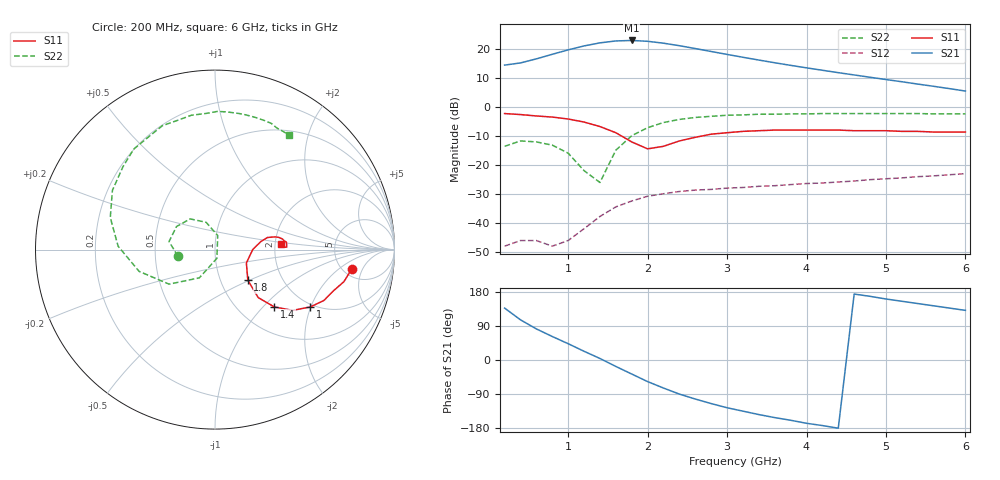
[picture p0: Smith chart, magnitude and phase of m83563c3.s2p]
!	MGA-83563 S PARAMETERS
!	Vd = 3 V L=4.7 nH  LAST UPDATED 10-15-97
# ghz	s ma r	50
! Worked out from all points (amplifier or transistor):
!   30 points, 200 MHz to 6 GHz, reference 50 ohm
!   highest |S21| = 22.9 dB at 1.8 GHz (marker M1)
!   |S21| within 3 dB of that: 1.036 GHz to 2.642 GHz (1.606 GHz wide, 87.3 % of centre)
!   unconditionally stable (mu >= 1): start of sweep to end of sweep
!   at 1.2 GHz: K = 3.89, MAG = 22.6 dB, |S12| = -41.9 dB
!   at 3.2 GHz: K = 1.07, MAG = 20.9 dB, |S12| = -27.7 dB
!   at 6 GHz: K = 1.46, MAG = 10.2 dB, |S12| = -23.0 dB
!   S11 on the Smith chart (normalised r, x): 200 MHz: 6.00, -3.16; 1 GHz: 1.91, -1.99; 1.4 GHz: 1.43, -1.16; 1.8 GHz: 1.35, -0.49; 6 GHz: 2.16, +0.16
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0.2  0.77 -8.0  5.26 137.0  0.004 56.0  0.21 -170.0
0.4  0.74 -14.0  5.74 106.0  0.005 42.0  0.26 170.0
0.6  0.7 -19.0  6.74 82.0  0.005 41.0  0.25 149.0
0.8  0.67 -25.0  8.08 62.0  0.004 59.0  0.22 129.0
1  0.62 -31.0  9.63 43.0  0.005 91.0  0.16 108.0
1.2  0.55 -38.0  11.26 23.0  0.008 107.0  0.08 79.0
1.4  0.46 -44.0  12.72 4.0  0.013 109.0  0.05 -78.0
1.6  0.36 -48.0  13.72 -17.0  0.019 103.0  0.18 -119.0
1.8  0.25 -43.0  13.99 -37.0  0.024 94.0  0.32 -143.0
2  0.19 -23.0  13.53 -57.0  0.029 85.0  0.44 -164.0
2.2  0.21 0.0  12.55 -74.0  0.032 77.0  0.54 178.0
2.4  0.26 10.0  11.36 -90.0  0.035 70.0  0.61 163.0
2.6  0.3 13.0  10.15 -103.0  0.037 65.0  0.66 150.0
2.8  0.34 12.0  9.03 -115.0  0.038 61.0  0.69 138.0
3  0.36 11.0  8.04 -126.0  0.04 57.0  0.72 129.0
3.2  0.38 9.0  7.18 -135.0  0.041 54.0  0.73 120.0
3.6  0.4 6.0  5.78 -152.0  0.044 50.0  0.75 106.0
4  0.4 4.0  4.72 -167.0  0.048 46.0  0.76 94.0
4.2  0.4 3.0  4.29 -173.0  0.049 44.0  0.77 89.0
4.6  0.39 2.0  3.56 174.0  0.053 40.0  0.77 80.0
5.2  0.38 2.0  2.72 155.0  0.06 34.0  0.77 69.0
6  0.37 5.0  1.88 131.0  0.071 26.0  0.76 57.0
